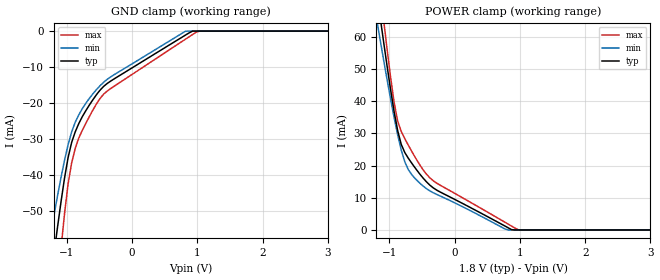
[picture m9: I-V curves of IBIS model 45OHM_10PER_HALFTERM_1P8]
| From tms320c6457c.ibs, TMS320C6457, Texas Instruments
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|   Model Cell 45OHM_10PER_HALFTERM_1P8
|45OHM_10PER_HALFTERM_1P8
[Model]   45OHM_10PER_HALFTERM_1P8
Model_type   Input
Polarity   Non-Inverting
Vinl =  0.8
Vinh =  1
C_comp   1.89p   1.72p   2.18p
[Model Spec]
Vinl   0.8   0.71   0.89
Vinh   1   0.91   1.09
D_overshoot_high 2.34 NA NA
D_overshoot_low -0.54 NA NA
D_overshoot_time 0.56n NA NA
S_overshoot_high 2.2 NA NA
S_overshoot_low -0.4 NA NA
[Receiver Thresholds]
Vth = 0.9V
Vth_min = 0.855V
Vth_max = 0.945V
Vinl_dc = -125mV
Vinh_dc = +125mV
Vinl_ac = -250mV
Vinh_ac = +250mV
Tslew_ac = 5.000ns
Threshold_sensitivity = 0.50
Reference_supply Pullup_ref
[Temperature Range]   25   125   -40
[Voltage Range]   1.8   1.62   1.98
[Pullup reference]   1.8   1.62   1.98
[POWER_clamp]
|   voltage   I(typ)   I(min)   I(max)
-1.8V     167.2mA    142.2mA    196.4mA
-1.2V     74.86mA    66.17mA    85.16mA
-1.145V   66.8mA     59.62mA    75.38mA
-1.091V   58.86mA    53.18mA    65.77mA
-1.036V   51.13mA    46.88mA    56.44mA
-927.3mV  36.8mA     34.94mA    39.67mA
-818.2mV  26.61mA    24.85mA    30.6mA
-654.5mV  20.69mA    17.13mA    24.35mA
-381.8mV  13.98mA    12.17mA    16.25mA
763.6mV   1.302mA    386.5uA    2.489mA
981.8mV   0A         0A         0A
3.6V      0A         0A         0A
[GND_clamp]
|   voltage   I(typ)   I(min)   I(max)
-1.8V     -155.3mA   -120.7mA   -211.3mA
-1.255V   -70.14mA   -57.31mA   -93.47mA
-1.145V   -54.88mA   -46.07mA   -71.34mA
-1.091V   -47.66mA   -40.85mA   -60.75mA
-1.036V   -40.97mA   -35.98mA   -50.89mA
-981.8mV  -35.25mA   -31.65mA   -42.59mA
-872.7mV  -28.08mA   -25.4mA    -32.7mA
-545.5mV  -17.68mA   -16.27mA   -20.24mA
-381.8mV  -14.57mA   -13.43mA   -16.69mA
818.2mV   -1.106mA   -33.07uA   -2.245mA
1.036V    0A         0A         0A
3.6V      0A         0A         0A
